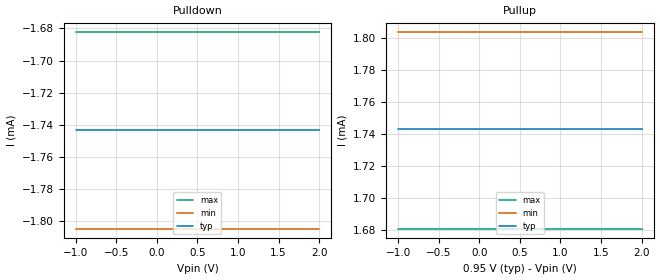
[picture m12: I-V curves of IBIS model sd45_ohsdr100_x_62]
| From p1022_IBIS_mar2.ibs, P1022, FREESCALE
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[Model]   sd45_ohsdr100_x_62
Model_type 3-state
Enable Active-High
Polarity Non-Inverting
|   TYP   MIN   MAX
C_comp   0.00pF   0.00pF   0.00pF
[Model Spec]
Vmeas   0.475   0.425   0.605
[Temperature Range] 65   125   -40
[Voltage Range]   0.95   0.85   1.21
[Pullup]
|   Vout(V)   TYP   WCS   BCS
-1V       1.743mA    1.803mA    1.681mA
2V        1.743mA    1.803mA    1.681mA
[Pulldown]
|   Vout(V)   TYP   WCS   BCS
-1V       -1.743mA   -1.805mA   -1.682mA
2V        -1.743mA   -1.805mA   -1.682mA
[GND Clamp]
|   Vout(V)   TYP   WCS   BCS
-1V       0A         0A         0A
1V        0A         0A         0A
[POWER Clamp]
|   Vout(V)   TYP   WCS   BCS
-1V       0A         0A         0A
0V        0A         0A         0A
[Ramp]
R_load=50
dV/dt_r  1.4958e-01/6.4236e-11  1.3455e-01/6.5371e-11  1.9119e-01/6.5914e-11
dV/dt_f  1.4958e-01/6.5678e-11  1.3454e-01/6.7506e-11  1.9120e-01/6.6813e-11
|[End   sd45_ohsdr100_x_62
